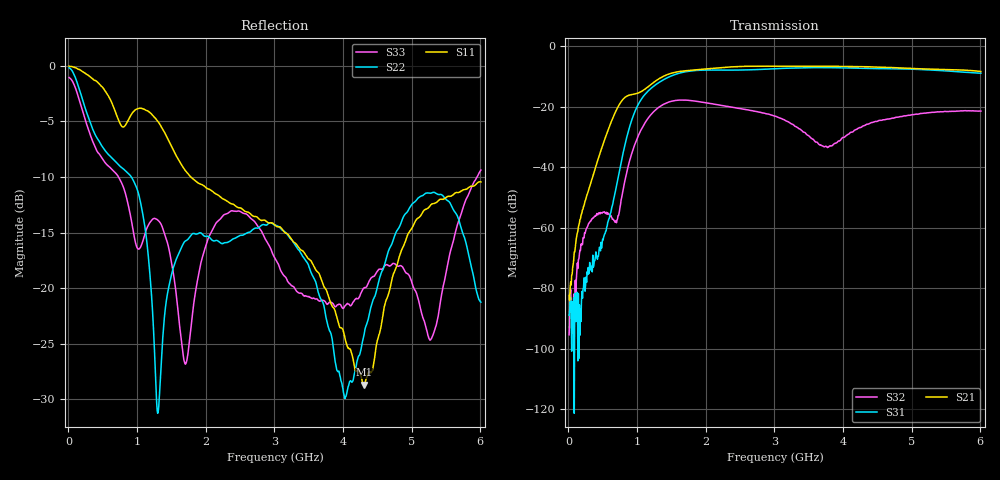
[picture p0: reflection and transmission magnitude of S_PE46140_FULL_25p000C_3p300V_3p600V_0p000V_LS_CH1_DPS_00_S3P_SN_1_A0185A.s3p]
! Device ID: PE46140_FULL
! File Path: z:\PE46140\MajorStates\25p000C\3p300\LS_CH1_DPS_00\PE46140_FULL_25p000C_3p300V_3p600V_0p000V_LS_CH1_DPS_00_S3P_SN_1_A0185A.s3p
! Serial: 1
! Lot: A0185A
! Temp: 25.000C
! VDD: 3.300
! VSS: 0.000
! Control_Hi: 3.600
! Control_Lo: 0.000
! Logic State: LS_CH1_DPS_00
! Port 1: RFIN
! Port 2: RFOUT1
! Port 3: RFOUT2
! ThroughPath:1-2
! IDD: 0.0003111135
! ISS: -1.644e-007
! Comment:
#  Hz  S  RI  R  50
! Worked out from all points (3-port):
!   801 points, 10 MHz to 6.01 GHz, reference 50 ohm
!   strongest paths, dB at 10 MHz, 1.51 GHz, 3.01 GHz, 4.51 GHz, 6.01 GHz:
!     S21: -82.3, -8.8, -6.6, -6.9, -8.3
!     S31: -88.8, -9.7, -7.4, -7.4, -8.9
!     S32: -95.3, -18.1, -23.1, -24.6, -21.4
!   lowest |S11| = -28.7 dB at 4.308 GHz (marker M1), VSWR 1.08, Z = 46.5 + j0.664 ohm
!   |S11| at or under -10 dB: 1.781 GHz to end of sweep
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1e7  0.9924 -0.0706  -7.38e-06 3.32e-05  -2.4e-05 9.44e-06
     2.17e-05 7.32e-05  0.9748 -0.0927  2.69e-05 -5.38e-06
     2.25e-05 -2.83e-05  1.68e-05 -2.84e-06  0.8808 -0.083
1.45e8  0.5429 -0.7954  -0.000859 0.000454  5.61e-05 -3.23e-05
        -0.000918 0.000476  0.2596 -0.765  -0.000274 0.000117
        -7.23e-05 3.81e-05  -0.000294 5.97e-05  0.2358 -0.6837
3.325e8  -0.3244 -0.8234  -0.00584 0.000755  -0.000102 0.000203
         -0.0058 0.000747  -0.4382 -0.3155  -0.000392 0.0013
         -4.24e-05 0.000212  -0.000373 0.00129  -0.3866 -0.2764
7.975e8  -0.5276 -0.0521  -0.0228 0.1325  0.0173 -0.00291
         -0.0228 0.1325  0.0989 0.3296  -0.00129 0.00426
         0.0172 -0.0029  -0.00125 0.0042  0.0941 0.2702
1.405e9  -0.3429 0.362  0.3207 -0.0705  -0.1429 0.2508
         0.321 -0.0701  -0.0244 0.0737  -0.0672 0.0908
         -0.1433 0.2509  -0.0673 0.0907  0.1539 -0.0817
1.975e9  -0.1291 0.2577  -0.118 -0.4036  0.4007 -0.0568
         -0.118 -0.4039  0.151 0.0818  0.0488 -0.1078
         0.401 -0.0568  0.049 -0.1079  0.0515 0.136
3.01e9  0.00704 0.1918  -0.2247 0.412  -0.3708 -0.2113
        -0.2256 0.4119  0.1825 -0.0585  0.0378 0.0589
        -0.371 -0.2116  0.0379 0.059  0.1266 -0.0498
4.3075e9  -0.0361 0.00712  0.39 -0.249  0.21 0.3797
          0.3905 -0.2486  0.0535 0.0306  0.0401 0.0281
          0.2103 0.3793  0.0401 0.0279  0.0974 -0.0239
5.215e9  -0.1534 -0.1666  -0.3077 -0.2888  0.3352 -0.2368
         -0.3072 -0.2894  0.2672 -0.0117  -0.0748 -0.0264
         0.3353 -0.2359  -0.0748 -0.0262  0.0606 -0.0249
6.01e9  -0.2505 -0.1656  -0.2205 0.3143  -0.1638 -0.3193
        -0.2206 0.3149  0.0856 -0.0121  0.0359 0.0769
        -0.1649 -0.3201  0.0359 0.0772  0.3171 0.1214
